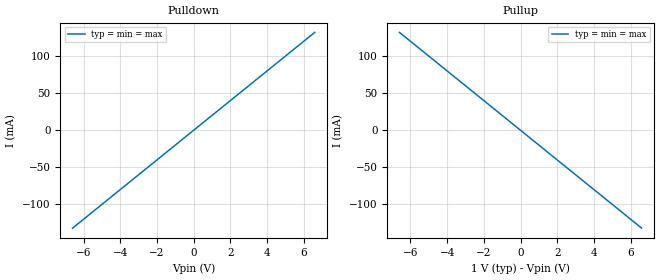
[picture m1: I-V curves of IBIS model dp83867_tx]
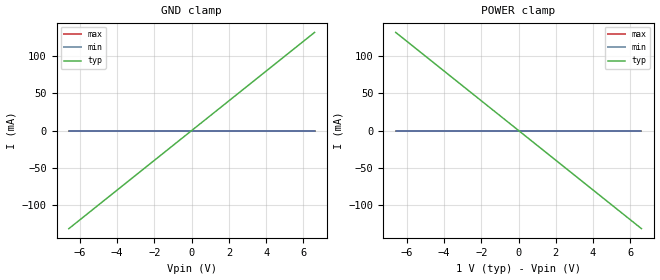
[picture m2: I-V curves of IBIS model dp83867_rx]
[IBIS Ver]   5.1
[File Name]   dp83867.ibs
[File Rev]   1.0
[Component]   dp83867
[Manufacturer] My Company
[Package]
R_pkg  0.0   NA   NA
L_pkg  0.0   NA   NA
C_pkg  0.0   NA   NA
[Pin]   signal_name   model_name   R_pin L_pin  C_pin
1p   dp83867_tx_p   dp83867_tx
1n   dp83867_tx_n   dp83867_tx
2p   dp83867_rx_2p   dp83867_rx
2n   dp83867_rx_2n   dp83867_rx
[Diff_Pin] inv_pin vdiff tdelay_typ tdelay_min tdelay_max
1p   1n   NA   NA   NA   NA
2p   2n   NA   NA   NA   NA
| Models and submodels in the file (2): dp83867_tx (Output), dp83867_rx (Input)
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[Model] dp83867_tx
Model_type Output
C_comp 0p 0p 0p
Cref = 0
Vref = 0.5
Rref = 50
Vmeas = 0.5
[Temperature_Range] 25 125 0
[Voltage Range] 1.0 1.0 1.0
[Algorithmic Model]
Executable Windows_cl16.00.40219.01_64 dp83867_TX_x64.dll dp83867_TX.ami
Executable Windows_cl16.00.40219.01_32 dp83867_TX.dll dp83867_TX.ami
|Executable Linux_gcc4.7.2_64 dp83867_TX_x64.so dp83867_TX.ami
[End Algorithmic Model]
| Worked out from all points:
|   slope of the pulldown table from 0 to 0.15 V, typ, clamps not added: 50 ohm
|   slope of the pullup table from 0 to 0.15 V, typ, clamps not added: 50 ohm
[Pulldown]
-6.6V     -132mA     -132mA     -132mA
0V        0A         0A         0A
6.6V      132mA      132mA      132mA
[Pullup]
-6.6V     132mA      132mA      132mA
0V        0A         0A         0A
6.6V      -132mA     -132mA     -132mA
[GND Clamp]
-6.6V     0A         0A         0A
0V        0A         0A         0A
6.6V      0A         0A         0A
[Power Clamp]
-6.6V     0A         0A         0A
0V        0A         0A         0A
6.6V      0A         0A         0A
[Ramp]
dV/dt_r 0.3/1.5p 0.3/1.5p 0.3/1.5p
dV/dt_f 0.3/1.5p 0.3/1.5p 0.3/1.5p
[Model] dp83867_rx
Model_type Input
C_comp 0p 0p 0p
Vinh = 0.25
Vinl = -0.25
[Temperature_Range] 25 125 0
[Voltage Range] 1.0 1.0 1.0
[Algorithmic Model]
Executable Windows_cl16.00.40219.01_64 dp83867_RX1_x64.dll dp83867_RX1.ami
Executable Windows_cl16.00.40219.01_32 dp83867_RX1.dll dp83867_RX1.ami
|Executable Linux_gcc4.7.2_64 dp83867_RX_x64.so dp83867_RX.ami
[End Algorithmic Model]
[GND Clamp]
-6.6V     -132mA     0A         0A
0V        0A         0A         0A
6.6V      132mA      0A         0A
[Power Clamp]
-6.6V     132mA      0A         0A
0V        0A         0A         0A
6.6V      -132mA     0A         0A
